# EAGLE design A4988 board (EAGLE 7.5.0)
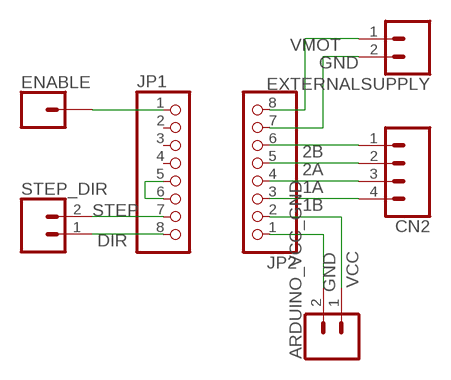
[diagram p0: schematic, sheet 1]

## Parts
ARDUINO_VCC_GND  CONN_02  [1X02]
CN2  CONN_04  [1X04]
ENABLE  CONN_01  [1X01]
EXTERNALSUPPLY  CONN_02  [1X02]
JP1  PINHD-1X8CLEANBIG  [1X08-CLEANBIG]
JP2  PINHD-1X8CLEANBIG  [1X08-CLEANBIG]
STEP_DIR  CONN_02  [1X02]

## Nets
1A: CN2.3 JP2.4
1B: CN2.4 JP2.3
2A: CN2.2 JP2.5
2B: CN2.1 JP2.6
DIR: JP1.8 STEP_DIR.1
GND: ARDUINO_VCC_GND.2 EXTERNALSUPPLY.2 JP2.1 JP2.7
N$1: ENABLE.1 JP1.1
N$12: JP1.5 JP1.6
STEP: JP1.7 STEP_DIR.2
VCC: ARDUINO_VCC_GND.1 JP2.2
VMOT: EXTERNALSUPPLY.1 JP2.8
Unconnected: JP1.2 JP1.3 JP1.4

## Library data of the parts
ARDUINO_VCC_GND EXTERNALSUPPLY STEP_DIR = SparkFun-Connectors:CONN_02: Multi connection point. Often used as Generic Header-pin footprint for 0.1 inch spaced/style header connections
CN2 = SparkFun-Connectors:CONN_04: Multi connection point. Often used as Generic Header-pin footprint for 0.1 inch spaced/style header connections On any of the 0.1 inch spaced packages, you can populate with these: Break Away Headers - Straight (PRT-00116) Break Away Male Headers - Right Angle (PRT-00553) Female Headers (PRT-00115)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; PROD_ID: CONN-09696
ENABLE = SparkFun-Connectors:CONN_01: Single connection point. Often used as Generic Header-pin footprint for 0.1 inch spaced/style header connections
JP1 JP2 = adafruit:PINHD-1X8: PIN HEADER

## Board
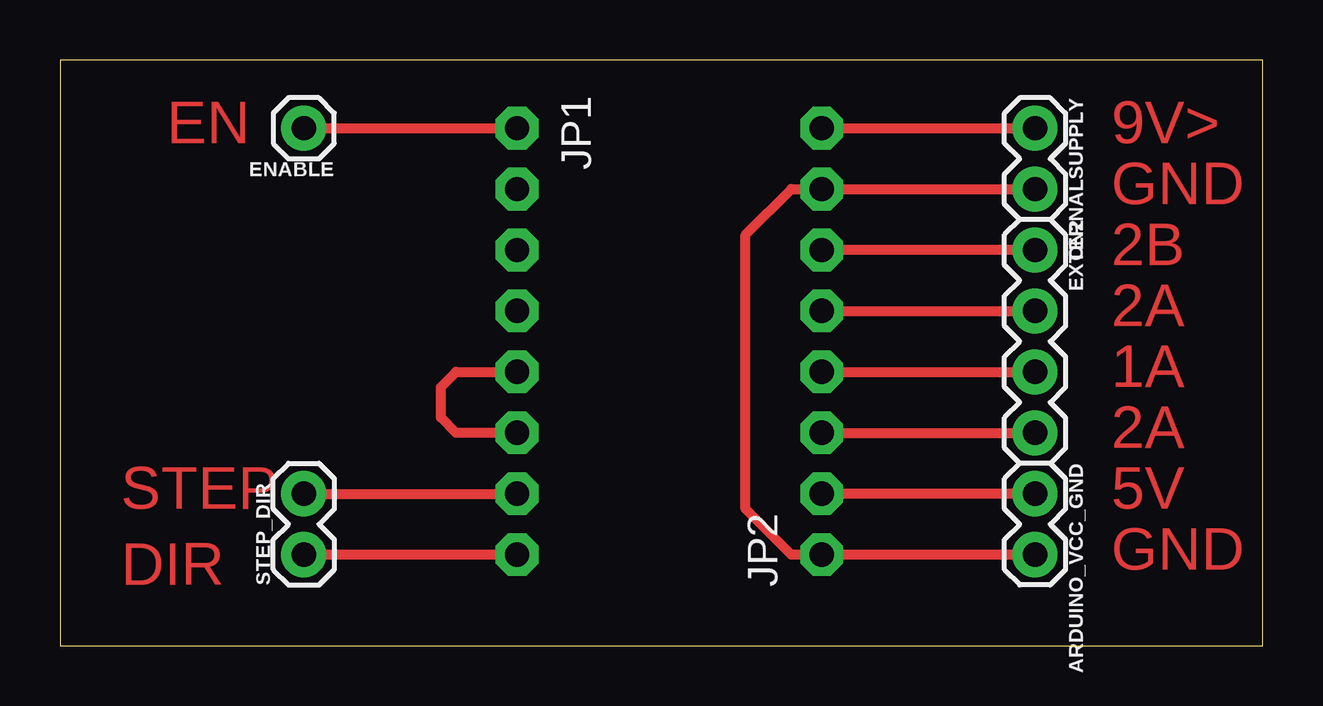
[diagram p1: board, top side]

Size 50.15 x 24.43 mm. Coordinates in mm from the lower left corner, seen from the top.
Outline: 0,0 50.15,0 50.15,24.43 0,24.43 0,0
Copper layers (1*16): Top 0.035mm / dielectric 1.5mm / Bottom 0.035mm
Design rules "default": minimum track width 10mil, minimum drill 24mil, track to track 8mil, track to pad 8mil, pad to pad 8mil, via to via 8mil, smd to smd 8mil, copper to edge 40mil, drill to drill 8mil, minimum pad ring 10mil, minimum via ring 8mil, stop-mask expansion 4mil, vias tented up to drill 0mil, thermal gap 10mil

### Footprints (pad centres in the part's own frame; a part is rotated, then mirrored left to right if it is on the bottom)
1X02 = drill 1.016 pad 1.88: 1 0,0; 2 2.54,0
1X04 = drill 1.016 pad 1.88: 1 0,0; 2 2.54,0; 3 5.08,0; 4 7.62,0
1X01 = drill 1.016 pad 1.88: 1 0,0
1X08-CLEANBIG = drill 1.016 pad 1.778 octagon: 1 -8.89,0; 2 -6.35,0; 3 -3.81,0; 4 -1.27,0; 5 1.27,0; 6 3.81,0; 7 6.35,0; 8 8.89,0

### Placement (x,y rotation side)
ARDUINO_VCC_GND  40.64,6.35 270 top
CN2  40.64,16.51 270 top
ENABLE  10.16,21.59 180 top
EXTERNALSUPPLY  40.64,21.59 270 top
JP1  19.05,12.7 270 top
JP2  31.75,12.7 90 top
STEP_DIR  10.16,3.81 90 top

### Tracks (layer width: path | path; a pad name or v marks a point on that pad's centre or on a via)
1A
  Top 0.406: JP2.4 CN2.3
1B
  Top 0.406: JP2.3 CN2.4
2A
  Top 0.406: JP2.5 CN2.2
2B
  Top 0.406: CN2.1 JP2.6
DIR
  Top 0.406: JP1.8 STEP_DIR.1
GND
  Top 0.406: EXTERNALSUPPLY.2 JP2.7 30.48,19.05 28.57,17.14 28.57,5.71 30.48,3.81 JP2.1 ARDUINO_VCC_GND.2
N$1
  Top 0.406: ENABLE.1 JP1.1
N$12
  Top 0.406: JP1.6 16.51,8.89 15.88,9.53 15.88,10.79 16.51,11.43 JP1.5
STEP
  Top 0.406: STEP_DIR.2 JP1.7
VCC
  Top 0.406: ARDUINO_VCC_GND.1 JP2.2
VMOT
  Top 0.406: JP2.8 EXTERNALSUPPLY.1

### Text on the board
Top: EN | 9V> | GND | 2B | 2A | 1A | 2A | STEP | 5V | DIR | GND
